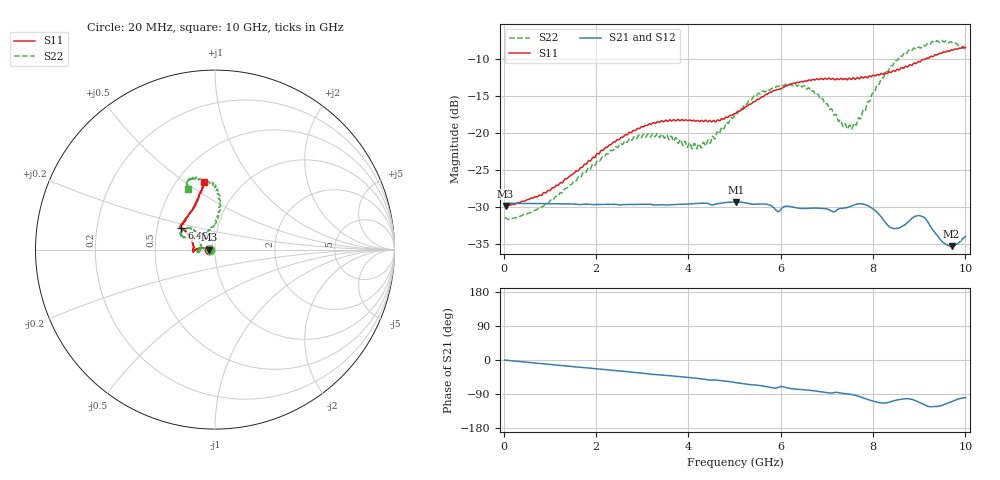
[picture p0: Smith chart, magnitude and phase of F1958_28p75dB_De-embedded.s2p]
! Integrated Device Technology
! Corporate Headquarters
! 6024 Silver Creek Valley Road
! San Jose, CA 95138  USA
! Phone:  1-408-284-8200
! Toll Free:  1-800-223-1366
! Webpage:  http://www.idt.com/
! Timing and RF Division
! 515 Groton Road, Suite 102
! Westford, MA 01886-6024
! Device:  F1958
! Description: 7-bit 0.25 dB Digital Step Attenuator
! Frequency:  0.001 -  6.000 GHz
! Package:  4x4 mm Thin QFN Plastic Package: 24 pin
! Ports:  2 RF, 12 DC
!  Pin  1  = D0
!  Pin  2  = VDD
!  Pin  3  = VMODE
!  Pin  4  = GND
!  Pin  5  = RF1  =  Port 1
!  Pin  6  = GND
!  Pin  7  = GND
!  Pin  8  = GND
!  Pin  9  = GND
!  Pin 10  = GND
!  Pin 11  = GND
!  Pin 12  = GND
!  Pin 13  = GND
!  Pin 14  = RF2  =  Port 2
!  Pin 15  = GND
!  Pin 16  = LE
!  Pin 17  = CLK
!  Pin 18  = DATA
!  Pin 19  = D6
!  Pin 20  = D5
!  Pin 21  = D4
!  Pin 22  = D3
!  Pin 23  = D2
!  Pin 24  = D1
! State:  115
! Atten State:  28.75 dB
! Voltage:  +3.30 Volts
! Current:  0.258 mA
! Data:  The device was measured on a F1958 evaluation board which has
!  individual transmission lines to the RF pins.  Data was collected
!  using a calibrated network analyzer.  The evaluation board was
!  de-embedded using Automatic Fixture Removal (AFR).
!  The reference plane is the edge of the package pin.
! Misc:
!  Action Tracker AT0419
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# GHz S dB R 50
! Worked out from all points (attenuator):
!   500 points, 20 MHz to 10 GHz, reference 50 ohm
!   highest |S21| = -29.31 dB at 5.04 GHz (marker M1); lowest = -35.3 dB at 9.7 GHz (marker M2)
!   lowest |S11| = -29.9 dB at 40 MHz (marker M3), VSWR 1.07, Z = 46.9 - j0.0416 ohm
!   |S11| at or under -10 dB: start of sweep to 9.132 GHz
!   |S22| runs from -31.7 to -7.5 dB; largest |S21 - S12| = 0.0003
!   S11 on the Smith chart (normalised r, x): 20 MHz: 0.94, -0.00; 6.42 GHz: 0.67, +0.17; 10 GHz: 0.67, +0.59
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0.02  -29.85 -178.9  -29.52 -0.2  -29.52 -0.2  -31.49 -179.0
0.04  -29.88 -179.2  -29.51 -0.4  -29.51 -0.3  -31.46 -178.5
0.84  -28.28 171.0  -29.55 -9.8  -29.54 -9.9  -29.97 171.9
1.7  -24.67 170.9  -29.65 -19.6  -29.65 -19.6  -25.58 170.7
2.62  -20.30 176.8  -29.69 -30.1  -29.66 -30.2  -21.08 179.7
3.36  -18.55 -176.0  -29.71 -39.1  -29.72 -39.1  -20.42 -170.2
4.24  -18.46 -179.4  -29.50 -49.1  -29.52 -49.2  -21.50 168.0
5.02  -17.38 160.5  -29.32 -59.4  -29.33 -59.4  -17.30 137.8
5.04  -17.27 159.5  -29.31 -59.8  -29.33 -59.8  -17.31 138.7
5.6  -15.11 150.6  -29.60 -68.2  -29.61 -68.2  -14.40 139.8
5.94  -14.10 148.1  -30.63 -72.5  -30.64 -72.4  -13.70 148.3
6.42  -13.09 147.4  -30.20 -77.8  -30.21 -77.8  -13.46 156.8
6.68  -12.80 146.5  -30.15 -80.6  -30.18 -80.6  -14.35 157.3
7.5  -12.63 138.1  -29.96 -90.2  -29.96 -90.0  -18.94 119.3
7.68  -12.58 135.2  -29.57 -95.5  -29.57 -95.5  -17.98 99.3
7.9  -12.38 128.8  -29.86 -104.7  -29.85 -104.8  -15.72 89.2
8.34  -11.76 118.7  -32.57 -111.7  -32.58 -112.0  -11.51 84.0
8.56  -11.49 115.1  -32.81 -104.6  -32.79 -104.7  -9.80 86.3
9.04  -10.26 106.7  -31.24 -113.8  -31.25 -113.9  -8.47 97.4
9.5  -9.13 101.2  -34.70 -119.2  -34.77 -119.2  -7.49 108.8
9.7  -8.74 100.4  -35.30 -110.2  -35.25 -109.6  -7.67 111.9
10  -8.42 99.6  -33.97 -99.4  -34.07 -99.3  -8.62 113.9
